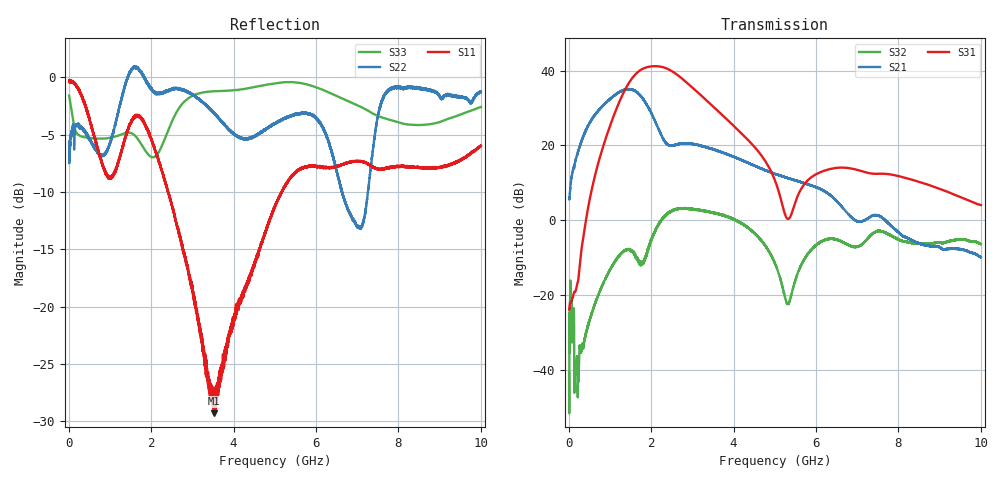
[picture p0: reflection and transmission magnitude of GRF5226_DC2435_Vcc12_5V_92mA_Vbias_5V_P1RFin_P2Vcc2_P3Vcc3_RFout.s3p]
!Keysight Technologies,N5245B,MY56052315,A.20.20.05
!Date: Friday, August 21, 2026 14:52:53
!Correction: S11(C  3-Port  )
!S12(C  3-Port  )
!S13(C  3-Port  )
!S21(C  3-Port  )
!S22(C  3-Port  )
!S23(C  3-Port  )
!S31(C  3-Port  )
!S32(C  3-Port  )
!S33(C  3-Port  )
!S3P File: Measurements: <S11,S12,S13>,
!<S21,S22,S23>,
!<S31,S32,S33>:
# Hz S  dB  R 50
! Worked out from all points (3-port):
!   9991 points, 10 MHz to 10 GHz, reference 50 ohm
!   strongest paths, dB at 10 MHz, 2.507 GHz, 5.005 GHz, 7.503 GHz, 10 GHz:
!     S31: -23.9, 39.8, 10.6, 12.4, 4.1
!     S21: 5.9, 19.9, 12.4, 1.3, -9.9
!     S32: -40.8, 2.5, -11.5, -2.9, -6.4
!   lowest |S11| = -29.3 dB at 3.518 GHz (marker M1), VSWR 1.07, Z = 49.4 + j3.34 ohm
!   |S11| at or under -10 dB: 2.409729 GHz to 2.410628 GHz (898.2 kHz wide, 0.0373 % of centre); 2.412 GHz to 5.167 GHz (2.755 GHz wide, 72.7 % of centre); 5.167164 GHz to 5.16853 GHz (1.366 MHz wide, 0.0264 % of centre)
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1e7  -0.39 -1.9  -52.15 26.2  -55.55 41.4
     5.92 51.0  -5.58 -51.8  -60.89 117.7
     -23.89 -150.2  -40.76 51.0  -1.59 -56.6
6.69e8  -5.83 -99.1  -40.72 103.3  -74.59 94.6
        28.60 24.8  -6.39 170.0  -40.87 -62.5
        13.29 7.6  -21.32 -1.8  -5.33 -172.4
1.189e9  -7.54 -109.3  -37.65 89.6  -59.45 92.7
         33.95 -34.2  -3.22 -161.1  -29.79 -135.8
         30.61 -58.5  -9.95 -75.0  -5.10 -175.2
1.535e9  -3.68 -143.7  -34.55 90.4  -56.61 87.3
         34.98 -90.1  0.80 179.6  -25.79 164.0
         37.90 -123.9  -8.09 -157.8  -4.89 179.5
1.885e9  -4.35 162.5  -32.92 76.4  -56.00 67.9
         31.06 -148.2  -0.34 149.8  -28.80 109.0
         40.86 166.3  -9.15 31.0  -6.52 179.1
2.295e9  -8.58 115.6  -33.37 72.5  -56.49 60.9
         21.67 -170.5  -1.32 138.5  -32.62 111.1
         40.88 96.1  0.62 -77.1  -5.68 -161.2
2.724e9  -14.14 76.5  -33.03 81.1  -56.50 73.8
         20.45 -155.3  -1.04 128.6  -29.16 96.0
         38.09 33.2  3.11 -145.5  -2.44 -166.7
3.518e9  -29.31 98.8  -29.47 88.7  -56.22 64.7
         18.88 172.8  -3.05 129.5  -29.00 48.2
         30.28 -44.5  1.86 138.7  -1.21 170.1
5.005e9  -11.32 167.8  -26.49 68.3  -55.44 66.1
         12.39 121.8  -4.03 109.1  -36.08 -22.2
         10.59 -133.9  -11.53 36.8  -0.52 155.8
1e10  -5.97 105.3  -26.13 38.0  -55.41 20.8
      -9.89 51.3  -1.25 88.0  -30.05 -11.3
      4.05 132.9  -6.42 -30.7  -2.59 71.1
